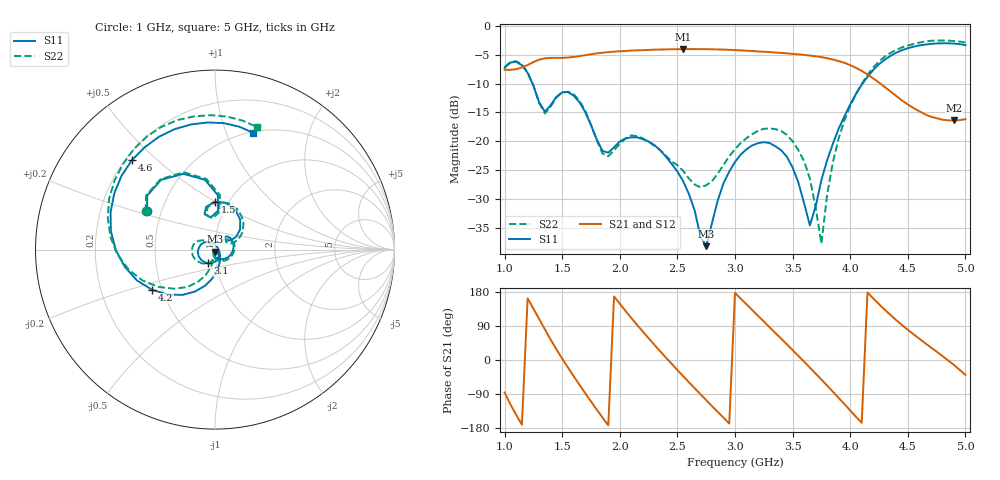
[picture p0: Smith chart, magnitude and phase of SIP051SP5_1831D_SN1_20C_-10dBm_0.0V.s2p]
# GHz  S  dB  R  50
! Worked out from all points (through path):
!   81 points, 1 GHz to 5 GHz, reference 50 ohm
!   highest |S21| = -3.97 dB at 2.55 GHz (marker M1); lowest = -16.4 dB at 4.9 GHz (marker M2)
!   lowest |S11| = -38.2 dB at 2.75 GHz (marker M3), VSWR 1.02, Z = 50.3 - j1.2 ohm
!   |S11| at or under -10 dB: 1.242 GHz to 4.106 GHz (2.864 GHz wide, 107 % of centre)
!   |S22| runs from -37.8 to -2.5 dB; largest |S21 - S12| = 0.0047
!   S11 on the Smith chart (normalised r, x): 1 GHz: 0.42, +0.22; 1.5 GHz: 0.87, +0.50; 3.1 GHz: 0.92, -0.14; 4.2 GHz: 0.44, -0.24; 4.6 GHz: 0.22, +0.42; 5 GHz: 0.51, +1.25
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1  -7.24 150.5  -7.58 -85.7  -7.58 -86.0  -7.10 151.2
1.2  -8.12 98.1  -6.74 162.6  -6.74 162.8  -8.03 97.0
1.35  -14.86 97.7  -5.59 80.6  -5.59 80.5  -15.15 94.5
1.5  -11.49 90.3  -5.51 3.4  -5.50 3.6  -11.53 88.3
1.7  -14.93 38.8  -5.04 -87.7  -5.04 -87.8  -14.72 32.4
1.95  -21.05 51.7  -4.43 167.7  -4.43 167.9  -21.58 42.6
2.15  -19.32 19.4  -4.20 92.6  -4.19 92.6  -19.11 5.3
2.35  -21.52 -31.3  -4.06 23.1  -4.06 23.1  -21.54 -46.4
2.55  -26.93 -84.8  -3.97 -42.5  -3.98 -42.5  -25.14 -85.7
2.75  -38.24 -77.1  -4.00 -105.9  -4.00 -106.0  -27.66 -96.6
3  -23.61 -88.2  -4.15 177.2  -4.14 177.3  -21.39 -116.3
3.1  -21.40 -117.0  -4.26 147.0  -4.26 146.7  -19.46 -134.3
3.35  -20.87 173.6  -4.58 71.3  -4.58 71.6  -17.89 175.6
3.65  -34.63 34.0  -5.11 -20.1  -5.11 -20.3  -26.46 130.7
3.7  -31.32 -25.8  -5.23 -36.0  -5.24 -35.6  -31.52 137.0
3.75  -26.75 -50.6  -5.38 -51.5  -5.40 -51.7  -37.80 -153.1
3.9  -17.82 -87.2  -6.07 -100.3  -6.07 -100.2  -19.49 -104.0
4.2  -7.61 -147.4  -9.08 162.4  -9.10 162.0  -7.15 -156.9
4.35  -5.15 -179.7  -11.34 118.8  -11.38 118.4  -4.63 173.0
4.6  -3.35 132.9  -14.79 56.2  -14.81 56.3  -2.85 128.8
4.9  -3.02 86.1  -16.38 -12.9  -16.38 -13.2  -2.57 84.7
5  -3.29 72.0  -16.16 -39.2  -16.14 -39.4  -2.83 71.0
